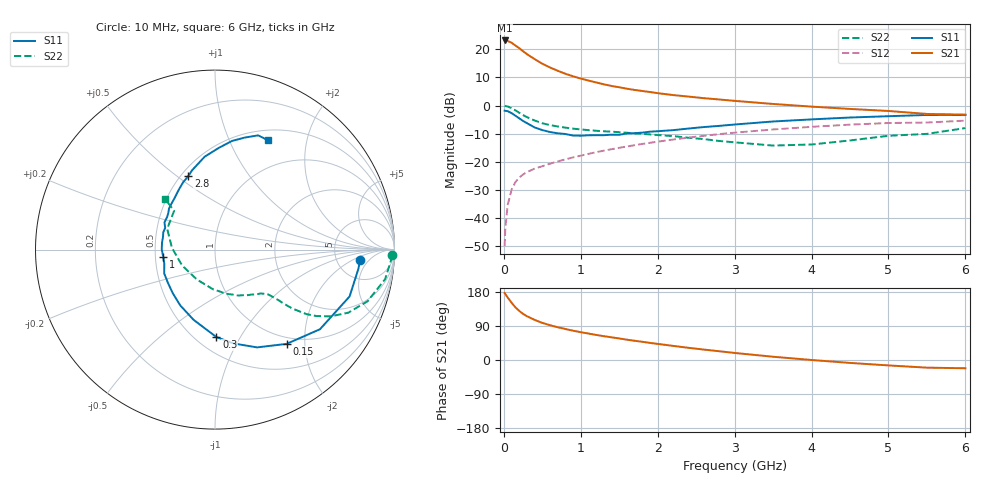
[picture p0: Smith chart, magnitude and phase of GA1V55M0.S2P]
! Infineon Technologies  Discrete & RF Semiconductors
! BF775
! Si NPN RF Bipolar Junction Transistor in SOT23
! VCE = 1.5 V  IC = 5 mA
! Common Emitter S-Parameters:  May  1996
# GHz  S  MA  R  50
!  f  S11  S21  S12  S22
! GHz  MAG  ANG  MAG  ANG  MAG  ANG  MAG  ANG
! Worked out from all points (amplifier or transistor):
!   36 points, 10 MHz to 6 GHz, reference 50 ohm
!   highest |S21| = 23.1 dB at 10 MHz (marker M1)
!   |S21| within 3 dB of that: start of sweep to 212.7 MHz
!   unconditionally stable (mu >= 1): 756.7 MHz to 4.41 GHz; 5.128 GHz to end of sweep
!   at 250 MHz: K = 0.50, MSG = 21.9 dB, |S12| = -24.5 dB
!   at 1.4 GHz: K = 1.15, MAG = 8.8 dB, |S12| = -15.5 dB
!   at 6 GHz: K = 1.01, MAG = 0.5 dB, |S12| = -5.4 dB
!   S11 on the Smith chart (normalised r, x): 10 MHz: 8.56, -2.98; 150 MHz: 0.89, -1.65; 300 MHz: 0.62, -0.80; 1 GHz: 0.55, -0.05; 2.8 GHz: 0.54, +0.55; 6 GHz: 0.62, +1.40
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0.01  0.8114 -4.2  14.26 177.0  0.0032 85.7  0.9885 -1.9
0.02  0.8056 -7.8  14.02 173.8  0.0068 85.6  0.9808 -4.0
0.05  0.794 -19.2  13.94 164.9  0.0172 79.6  0.9618 -9.9
0.1  0.7341 -37.2  13.01 151.3  0.0319 70.9  0.8975 -18.7
0.15  0.6595 -52.8  11.6 139.1  0.0437 64.5  0.822 -25.3
0.2  0.5932 -66.7  10.43 129.6  0.0528 59.9  0.7444 -30.0
0.25  0.5332 -78.8  9.198 121.6  0.0597 56.5  0.6761 -33.2
0.3  0.4872 -89.1  8.157 115.5  0.066 55.0  0.6239 -35.2
0.4  0.4089 -107.0  6.656 105.9  0.0759 53.2  0.5421 -37.3
0.5  0.3665 -121.8  5.514 97.9  0.0837 52.9  0.4848 -38.2
0.6  0.3388 -133.8  4.729 91.8  0.093 53.1  0.4493 -38.6
0.7  0.3217 -144.3  4.137 86.5  0.102 53.5  0.4255 -39.1
0.8  0.3127 -154.9  3.659 81.8  0.1109 53.7  0.4054 -39.6
1  0.2915 -172.4  3.009 73.4  0.1291 54.4  0.3768 -40.9
1.1  0.2966 179.8  2.771 69.8  0.1387 54.6  0.3662 -42.2
1.6  0.3195 151.8  1.989 53.6  0.1878 52.9  0.3287 -49.5
2.2  0.3658 127.8  1.533 37.3  0.2491 48.5  0.287 -63.1
2.8  0.4355 110.0  1.28 23.1  0.3109 42.1  0.2352 -83.4
3.5  0.5211 96.3  1.066 8.6  0.376 33.3  0.1949 -121.0
4.5  0.6128 81.1  0.87 -7.7  0.4582 20.0  0.2401 177.6
5.5  0.6802 69.3  0.709 -20.2  0.4989 5.7  0.314 136.5
6  0.6772 64.3  0.69 -21.8  0.5397 1.7  0.3982 134.6
